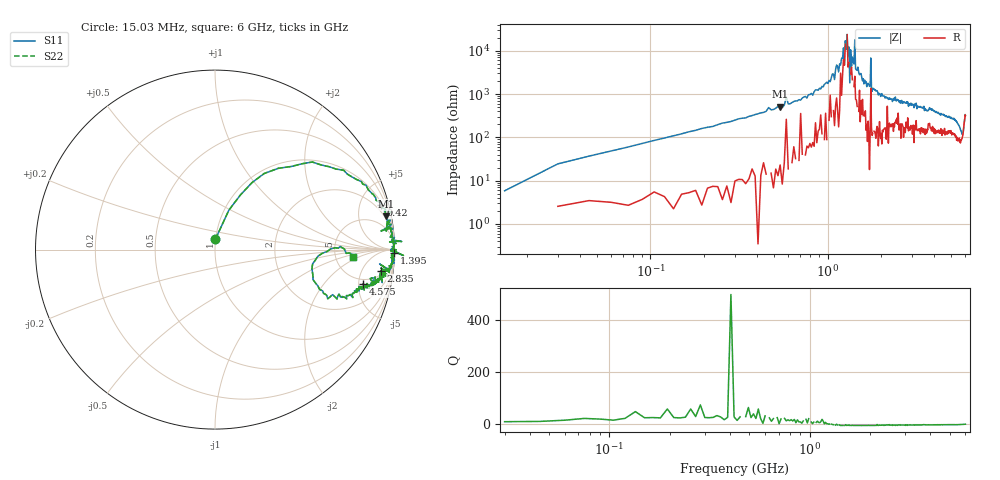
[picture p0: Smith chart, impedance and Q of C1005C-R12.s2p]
!	Network	Analyzer	HP8753E.07.74:	Oct	30	2002	Serial	No.	JP38451487
!	Hewlett-Packard
!	28	Aug	2009	9:23:40
!	Frequency	S11	S21	S12	S22
#	HZ	S	RI	R	50
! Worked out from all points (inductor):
!   400 points, 15.03 MHz to 6 GHz, reference 50 ohm
!   read as one part in series: L = 128 nH near 45.03 MHz
!   highest Q = 29 at 540 MHz (marker M1), where L = 150 nH
!   self-resonance near 1.26 GHz
!   S11 on the Smith chart (normalised r, x): 15.03 MHz: 1.00, +0.12; 420 MHz: 1.26, +7.37; 1.395 GHz: open; 2.835 GHz: 7, -12; 4.575 GHz: 4.22, -5.69; 6 GHz: 7.38, -1.42
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1.502992e7  0.00258 0.0583  0.997 -0.0583  0.997 -0.0583  0.00258 0.0583
9.002955e7  0.353 0.453  0.647 -0.453  0.647 -0.453  0.353 0.453
4.200279e8  0.924 0.248  0.0762 -0.248  0.0762 -0.248  0.924 0.248
5.400273e8  0.955 0.186  0.0451 -0.186  0.0451 -0.186  0.955 0.186
1.020025e9  0.992 0.0474  0.00803 -0.0474  0.00803 -0.0474  0.992 0.0474
1.245024e9  0.979 0  0.0211 0  0.0211 0  0.979 0
1.290024e9  0.996 -0.000641  0.00415 0.000641  0.00415 0.000641  0.996 -0.000641
1.335023e9  1.05 -0.0333  -0.0475 0.0333  -0.0475 0.0333  1.05 -0.0333
1.350023e9  0.997 -0.00909  0.00269 0.00909  0.00269 0.00909  0.997 -0.00909
1.395023e9  1 -0.0179  -0.00067 0.0179  -0.00067 0.0179  1 -0.0179
1.425023e9  0.999 -0.00558  0.000855 0.00558  0.000855 0.00558  0.999 -0.00558
1.440023e9  0.994 -0.0255  0.00583 0.0255  0.00583 0.0255  0.994 -0.0255
1.725021e9  0.995 -0.0661  0.00519 0.0661  0.00519 0.0661  0.995 -0.0661
1.755021e9  0.997 -0.0143  0.00314 0.0143  0.00314 0.0143  0.997 -0.0143
1.785021e9  0.985 -0.0841  0.0154 0.0841  0.0154 0.0841  0.985 -0.0841
2.01002e9  0.978 -0.0977  0.0225 0.0977  0.0225 0.0977  0.978 -0.0977
2.835016e9  0.923 -0.119  0.0767 0.119  0.0767 0.119  0.923 -0.119
3.015015e9  0.942 -0.152  0.0579 0.152  0.0579 0.152  0.942 -0.152
4.00501e9  0.885 -0.196  0.115 0.196  0.115 0.196  0.885 -0.196
4.575007e9  0.825 -0.191  0.175 0.191  0.175 0.191  0.825 -0.191
5.010005e9  0.802 -0.217  0.198 0.217  0.198 0.217  0.802 -0.217
6e9  0.768 -0.0393  0.232 0.0393  0.232 0.0393  0.768 -0.0393
